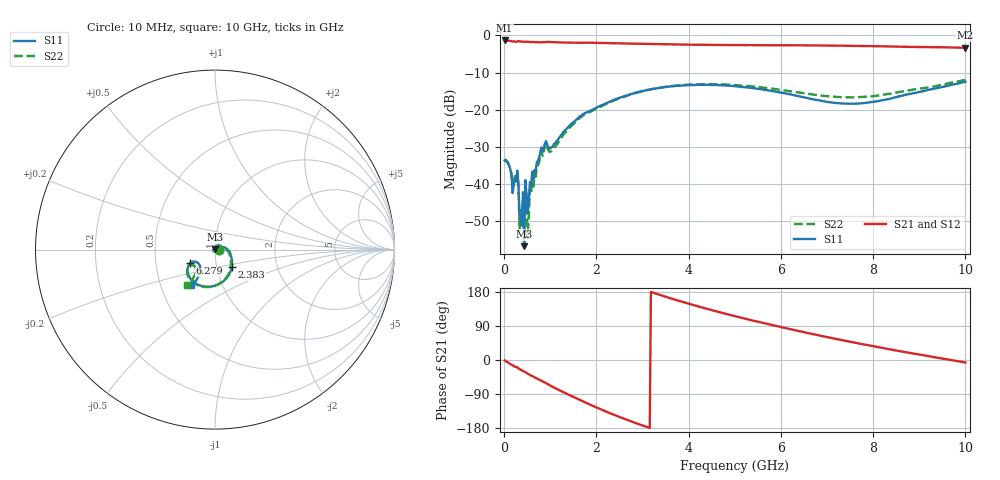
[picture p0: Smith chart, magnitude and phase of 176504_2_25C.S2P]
!  2-Port S-parameters saved by WinCal
! VAR MeasName=S-Parameters (CALIBRATED_DATA) read from VNA (N5242A)
! VAR MeasDate=2017-11-2 16:05:24
! VAR NAME=176504_2_25C
! VAR FILENAME=176504_2_25C.S2P
! VAR DATE=2017-11-2 16:05:24
! VAR PHYS_PORTS=2,3
# Hz S DB R 50
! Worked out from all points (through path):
!   401 points, 10 MHz to 10 GHz, reference 50 ohm
!   highest |S21| = -1.34 dB at 10 MHz (marker M1); lowest = -3.3 dB at 10 GHz (marker M2)
!   lowest |S11| = -56.7 dB at 434.6 MHz (marker M3), VSWR 1.00, Z = 49.9 + j0.0559 ohm
!   |S11| at or under -10 dB: start of sweep to end of sweep
!   |S22| runs from -54.5 to -12.0 dB; largest |S21 - S12| = 0.006
!   S11 on the Smith chart (normalised r, x): 10 MHz: 1.04, -0.00; 2.383 GHz: 1.18, -0.24; 6.279 GHz: 0.75, -0.12; 10 GHz: 0.72, -0.30
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1e7  -33.63 -3.3  -1.34 -0.9  -1.35 -0.9  -33.80 -2.9
8.4925e7  -34.22 -39.5  -1.41 -6.9  -1.41 -6.9  -34.37 -41.9
2.098e8  -39.99 -96.4  -1.58 -15.8  -1.58 -15.8  -39.22 -100.3
2.5975e8  -39.34 146.3  -1.71 -18.5  -1.71 -18.5  -39.16 153.0
3.84625e8  -51.20 -174.4  -1.66 -27.6  -1.66 -27.6  -48.32 -158.3
4.34575e8  -56.73 157.4  -1.67 -31.1  -1.66 -31.0  -53.16 -150.2
4.84525e8  -42.62 95.4  -1.71 -34.1  -1.71 -34.1  -44.58 103.9
5.095e8  -47.93 66.6  -1.68 -36.0  -1.68 -36.0  -54.46 68.2
5.5945e8  -39.45 85.5  -1.75 -39.1  -1.75 -39.1  -41.29 91.3
6.094e8  -36.66 85.4  -1.79 -42.3  -1.79 -42.3  -37.76 89.3
8.5915e8  -30.25 48.1  -1.84 -58.1  -1.84 -58.1  -31.16 46.1
1.033975e9  -30.09 23.3  -1.79 -69.7  -1.79 -69.7  -31.09 17.8
1.683325e9  -21.47 -10.4  -1.95 -107.7  -1.95 -107.7  -21.80 -13.9
2.382625e9  -17.33 -46.7  -2.08 -144.6  -2.08 -144.6  -17.47 -49.1
3.35665e9  -14.13 -86.3  -2.35 172.6  -2.36 172.6  -14.08 -87.1
4.180825e9  -13.28 -113.2  -2.50 142.3  -2.52 142.4  -13.14 -112.4
5.005e9  -13.65 -133.8  -2.58 115.7  -2.58 115.8  -13.34 -131.6
6.278725e9  -16.07 -151.4  -2.65 79.3  -2.64 79.4  -15.14 -147.2
6.678325e9  -17.13 -151.2  -2.65 68.8  -2.67 68.9  -15.86 -147.5
7.55245e9  -18.36 -138.1  -2.80 46.9  -2.80 46.9  -16.67 -139.5
8.35165e9  -17.07 -124.8  -2.95 28.3  -2.98 28.5  -15.70 -130.0
1e10  -12.48 -123.4  -3.31 -6.6  -3.32 -6.3  -11.95 -128.6
